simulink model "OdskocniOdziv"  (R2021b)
settings: Solver=ode45  StartTime=0.0  StopTime=0.01  MaxStep=1e-5  RelTol=1e-3  EnableMultiTasking=on
libraries: fl_lib x8, nesl_utility x3

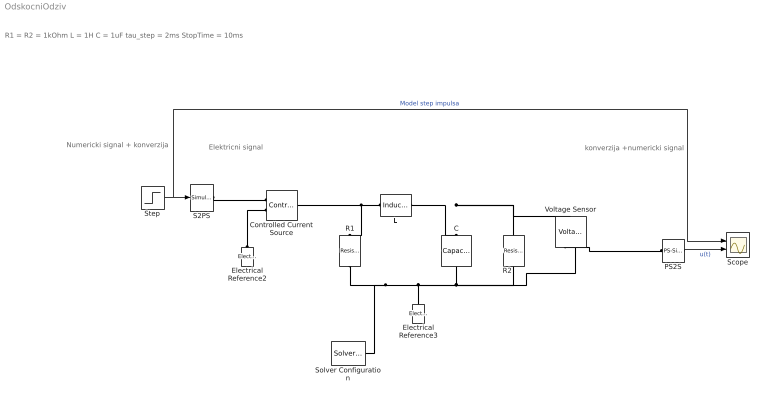
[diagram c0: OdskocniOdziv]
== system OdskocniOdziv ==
  note: R1 = R2 = 1kOhm L = 1H C = 1uF tau_step = 2ms StopTime = 10ms
  note: Elektricni signal
  note: konverzija +numericki signal
  note: Numericki signal + konverzija
  C : fl_lib/Electrical/Electrical Elements/Capacitor  c=1e-6 F  r=0 Ohm  g=0 1/Ohm  i_specify=off  i_priority=None  i=0 A  i_nominal_specify=off  i_nominal_unit=A  i_nominal_value=1  v_specify=off  v_priority=None  v=0 V  v_nominal_specify=off  v_nominal_unit=V  v_nominal_value=1  vc_specify=on  vc_priority=High  vc=0 V  vc_nominal_specify=off  vc_nominal_unit=V  vc_nominal_value=1
  Controlled Current Source : fl_lib/Electrical/Electrical Sources/Controlled Current Source
  Electrical Reference2 : fl_lib/Electrical/Electrical Elements/Electrical Reference
  Electrical Reference3 : fl_lib/Electrical/Electrical Elements/Electrical Reference
  L : fl_lib/Electrical/Electrical Elements/Inductor  l=1 H  r=0 Ohm  g=0 1/Ohm  i_specify=off  i_priority=None  i=0 A  i_nominal_specify=off  i_nominal_unit=A  i_nominal_value=1  v_specify=off  v_priority=None  v=0 V  v_nominal_specify=off  v_nominal_unit=V  v_nominal_value=1  i_L_specify=on  i_L_priority=High  i_L=0 A  i_L_nominal_specify=off  i_L_nominal_unit=A  i_L_nominal_value=1
  PS2S : nesl_utility/PS-Simulink Converter  PhysicalDomain=network_engine_domain  SubClassName=ps_output  LeftPortType=input  RightPortType=output  PseudoPeriodic=off  Frequencies=[]  Unit=1  AffineConversion=off
  R1 : fl_lib/Electrical/Electrical Elements/Resistor  R=1 kOhm  i_specify=off  i_priority=None  i=0 A  i_nominal_specify=off  i_nominal_unit=A  i_nominal_value=1  v_specify=off  v_priority=None  v=0 V  v_nominal_specify=off  v_nominal_unit=V  v_nominal_value=1
  R2 : fl_lib/Electrical/Electrical Elements/Resistor  R=1 kOhm  i_specify=off  i_priority=None  i=0 A  i_nominal_specify=off  i_nominal_unit=A  i_nominal_value=1  v_specify=off  v_priority=None  v=0 V  v_nominal_specify=off  v_nominal_unit=V  v_nominal_value=1
  S2PS : nesl_utility/Simulink-PS Converter  PhysicalDomain=network_engine_domain  SubClassName=ps_input  LeftPortType=input  RightPortType=output  PseudoPeriodic=off  Frequencies=[]  NoiseDistribution=none  NoiseParameters=[]  Unit=1  AffineConversion=off  FilteringAndDerivatives=zero  SimscapeFilterOrder=1  InputFilterTimeConstant=0.001  UdotUserProvided=1
  Scope : Scope  NumInputPorts=2
  Solver Configuration : nesl_utility/Solver Configuration  PhysicalDomain=network_engine_domain  SubClassName=solver  LeftPortType=input  RightPortType=generic  Tones=[]  Harmonics=[]  SimulateNoise=off  Profile=off  UseLocalSampling=off  EnableSwitchedLinearOptims=on  FrequencyDomain=off  UseCCode=off  RelTol=0.001  AbsTol=1e-06  MinStep=1e-09  ToWorkspace=off  RevertToSquareIcSolve=off  NumHomotopyIterations=100  PhasorMode=off  PhasorModeNumHarmonics=1  DoDC=off  ResidualTolerance=1e-09  UseLocalSolver=off  LocalSolverChoice=NE_BACKWARD_EULER_ADVANCER  LocalSolverSampleTime=0.001  DoFixedCost=off  MaxNonlinIter=3  MaxModeIter=2  ComputeImpulses=off  ImpulseIterations=2  LinearAlgebra=Sparse  EquationFormulation=NE_TIME_EF  DelaysMemoryBudget=1024  AutomaticFiltering=on  FilteringTimeConstant=0.001  PartitionStorageMethod=AS_NEEDED  PartitionMemoryBudget=1024  PartitionMethod=FAST
  Step : Step  Time=0.002  After=1e-3  SampleTime=0
  Voltage Sensor : fl_lib/Electrical/Electrical Sensors/Voltage Sensor
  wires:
  PS2S/1 -> Scope/2  "u(t)"
  Step/1 -> Scope/1, S2PS/1  "Model step impulsa"
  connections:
  L/LConn1 -- Controlled Current Source/LConn1 -- R1/LConn1
  L/RConn1 -- Voltage Sensor/LConn1 -- R2/LConn1 -- C/LConn1
  Voltage Sensor/RConn2 -- R2/RConn1 -- C/RConn1 -- Electrical Reference3/LConn1 -- Solver Configuration/RConn1 -- R1/RConn1
  PS2S/LConn1 -- Voltage Sensor/RConn1
  Electrical Reference2/LConn1 -- Controlled Current Source/RConn2
  S2PS/RConn1 -- Controlled Current Source/RConn1
